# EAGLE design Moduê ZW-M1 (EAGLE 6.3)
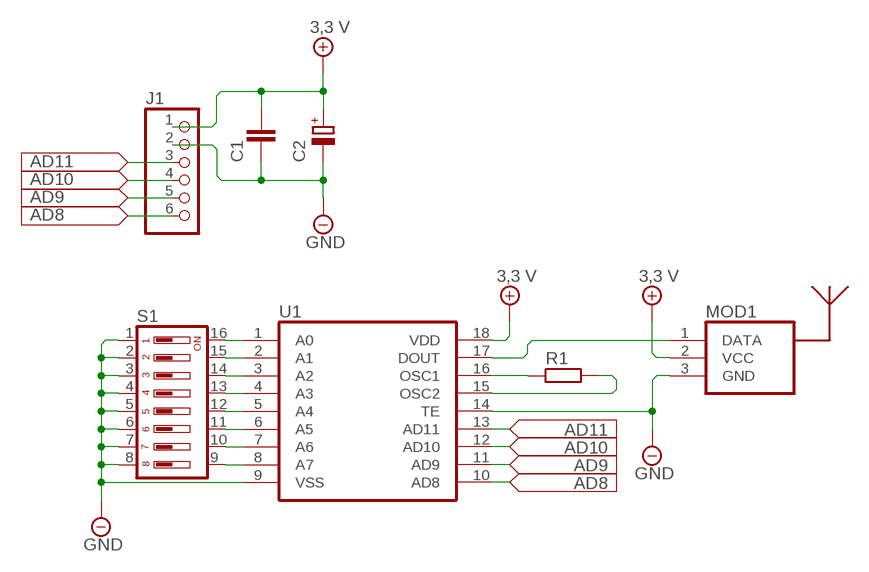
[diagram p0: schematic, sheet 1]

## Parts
C1  KONDENSATOR_CERAMICZNY  [KONDENSATOR_CERAMICZNY]
C2  KONDENSATOR_ELEKTROLITYCZNY_1  [KONDENSATOR_ELEKTROLITYCZNY_1]
J1  ZŁĄCZE_6_PIN  [ZŁĄCZE_6_PIN]
MOD1  NADAJNIK433MHZ  [NADAJNIK433MHZ]
R1  REZYSTOR  [REZYSTOR]
S1  DIP_SWITCH_8  [DIP_SWITCH_8]
U1  HT12F  [HT12F]

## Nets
5V: C1.1 C2.+ J1.1 MOD1.2(VCC) U1.18(VDD) ; supply symbol labelled 3,3 V
AD8: J1.6 U1.10(AD8)
AD9: J1.5 U1.11(AD9)
AD10: J1.4 U1.12(AD10)
AD11: J1.3 U1.13(AD11)
GND: C1.2 C2.- J1.2 MOD1.3(GND) S1.1 S1.2 S1.3 S1.4 S1.5 S1.6 S1.7 S1.8 U1.9(VSS) U1.14(TE)
N$18: S1.16 U1.1(A0)
N$22: S1.15 U1.2(A1)
N$23: S1.14 U1.3(A2)
N$24: S1.13 U1.4(A3)
N$25: S1.12 U1.5(A4)
N$26: S1.11 U1.6(A5)
N$27: S1.10 U1.7(A6)
N$28: S1.9 U1.8(A7)
N$29: R1.2 U1.15(OSC2)
N$30: R1.1 U1.16(OSC1)
N$35: MOD1.1(DATA) U1.17(DOUT)

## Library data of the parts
C1 = Własne:KONDENSATOR_CERAMICZNY
C2 = Własne:KONDENSATOR_ELEKTROLITYCZNY_1
J1 = Własne:ZŁĄCZE_6_PIN
MOD1 = Własne:NADAJNIK433MHZ
R1 = Własne:REZYSTOR
S1 = Własne:DIP_SWITCH_8
U1 = Własne:HT12F

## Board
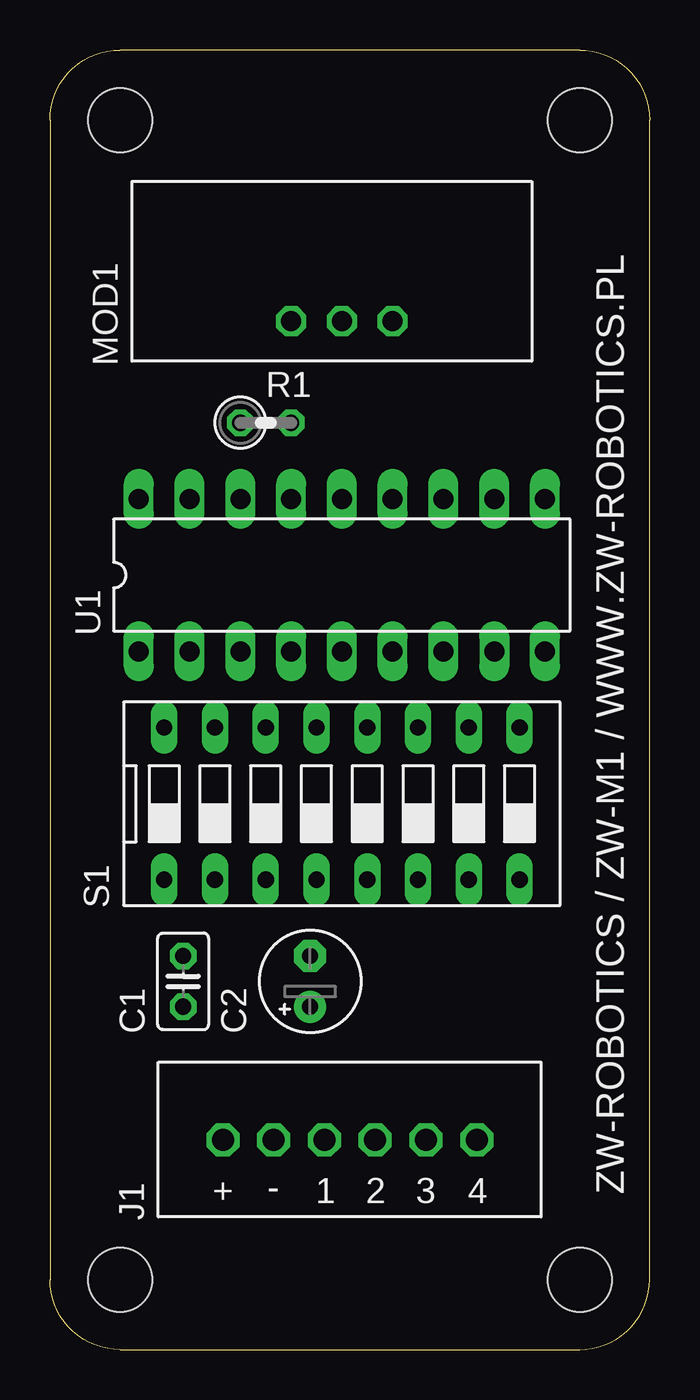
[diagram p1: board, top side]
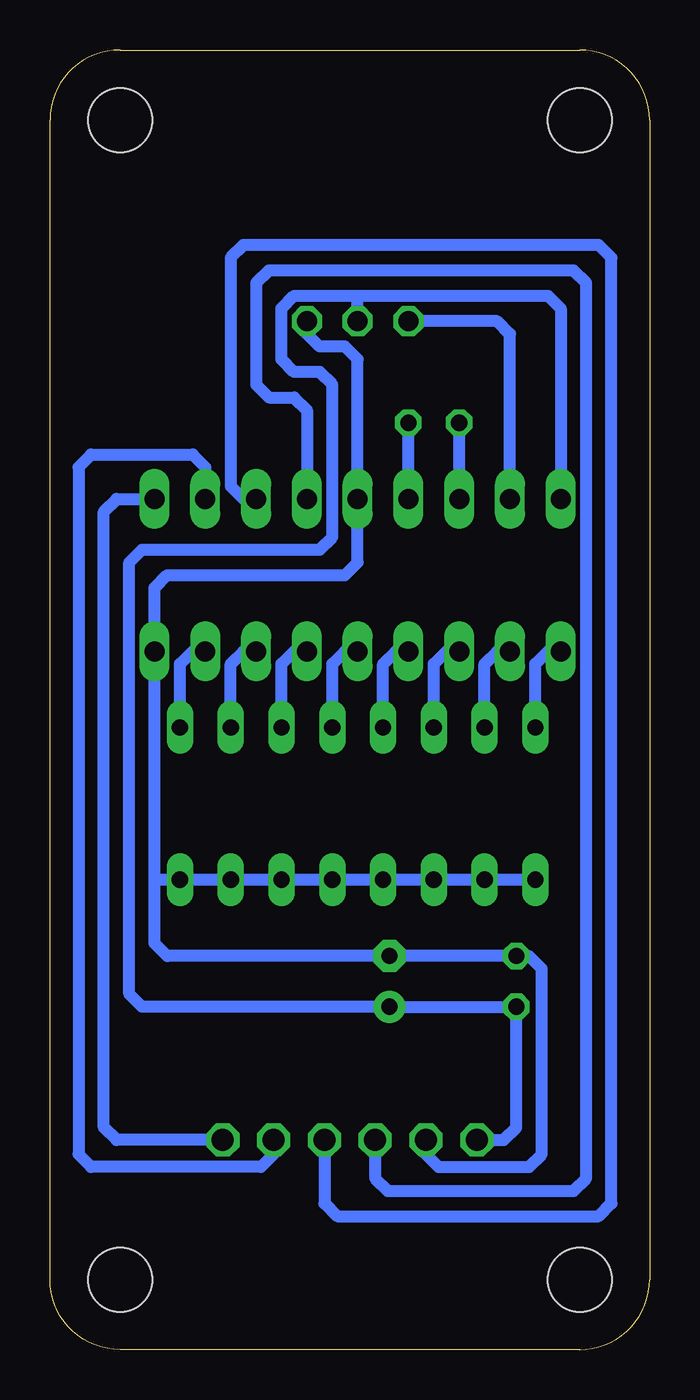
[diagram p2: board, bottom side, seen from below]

Size 30 x 65 mm. Coordinates in mm from the lower left corner, seen from the top.
Outline: 3.5,0 26.5,0 arc90 30,3.5 30,61.5 arc90 26.5,65 3.5,65 arc90 0,61.5 0,3.5 arc90 3.5,0
Copper layers (1*16): Top 0.035mm / dielectric 1.5mm / Bottom 0.035mm
Design rules "default": minimum track width 10mil, minimum drill 24mil, track to track 8mil, track to pad 8mil, pad to pad 8mil, via to via 8mil, smd to smd 8mil, copper to edge 40mil, drill to drill 8mil, minimum pad ring 10mil, minimum via ring 8mil, stop-mask expansion 4mil, vias tented up to drill 0mil, thermal gap 10mil
Holes 3.2 mm at 3.5,3.5 26.5,3.5 3.5,61.5 26.5,61.5

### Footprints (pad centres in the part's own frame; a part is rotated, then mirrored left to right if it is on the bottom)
KONDENSATOR_CERAMICZNY = drill 0.813 octagon: 1 -1.27,0; 2 1.27,0
KONDENSATOR_ELEKTROLITYCZNY_1 = drill 0.813 pad 1.6: + -1.27,0 | drill 0.813 pad 1.6 octagon: - 1.27,0
ZŁĄCZE_6_PIN = drill 1.1 octagon: 1 -6.35,0; 2 -3.81,0; 3 -1.27,0; 4 1.27,0; 5 3.81,0; 6 6.35,0
NADAJNIK433MHZ = drill 1 octagon: 1 -2.54,2.54; 2 -2.54,0; 3 -2.54,-2.54
REZYSTOR = drill 0.813 octagon: 1 -1.27,0; 2 1.27,0
DIP_SWITCH_8 = drill 0.813 long: 1 -8.89,-3.81; 2 -6.35,-3.81; 3 -3.81,-3.81; 4 -1.27,-3.81; 5 1.27,-3.81; 6 3.81,-3.81; 7 6.35,-3.81; 8 8.89,-3.81; 9 8.89,3.81; 10 6.35,3.81; 11 3.81,3.81; 12 1.27,3.81; 13 -1.27,3.81; 14 -3.81,3.81; 15 -6.35,3.81; 16 -8.89,3.81
HT12F = drill 1 long: 1 -10.16,-3.81; 2 -7.62,-3.81; 3 -5.08,-3.81; 4 -2.54,-3.81; 5 0,-3.81; 6 2.54,-3.81; 7 5.08,-3.81; 8 7.62,-3.81; 9 10.16,-3.81; 10 10.16,3.81; 11 7.62,3.81; 12 5.08,3.81; 13 2.54,3.81; 14 0,3.81; 15 -2.54,3.81; 16 -5.08,3.81; 17 -7.62,3.81; 18 -10.16,3.81

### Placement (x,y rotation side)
C1  6.67,18.41 90 top
C2  13.02,18.41 90 top
J1  15,10.48 0 top
MOD1  14.61,53.98 90 top
R1  10.79,46.35 0 top
S1  14.61,27.3 0 top
U1  14.61,38.73 0 top

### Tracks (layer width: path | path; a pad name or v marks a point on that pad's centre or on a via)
5V
  Bottom 0.61: J1.1 7.3,10.48 6.67,11.11 C1.1 C2.+ 25.4,17.14 26.04,17.78 26.04,39.37 25.4,40.01 16.51,40.01 15.88,40.64 15.88,48.26 16.51,48.9 17.78,48.9 18.41,49.53 18.41,52.07 17.78,52.7 14.61,52.7 | MOD1.2 14.61,52.7 | 14.61,52.7 5.08,52.7 4.45,52.07 U1.18
AD8
  Bottom 0.61: J1.6 26.67,10.48 27.3,11.11 27.3,41.91 26.67,42.55 U1.10
AD9
  Bottom 0.61: J1.5 18.81,9.77 19.45,9.13 27.94,9.13 28.57,9.77 28.57,44.13 27.94,44.77 22.86,44.77 22.23,44.13 U1.11
AD10
  Bottom 0.61: J1.4 16.27,7.3 15.63,6.67 2.54,6.67 1.91,7.3 1.91,54.61 2.54,55.24 20.32,55.24 20.95,54.61 20.95,43.18 20.32,42.55 U1.12
AD11
  Bottom 0.61: J1.3 13.73,8.57 13.1,7.94 3.81,7.94 3.17,8.57 3.17,53.34 3.81,53.98 19.05,53.98 19.68,53.34 19.68,48.26 19.05,47.62 17.78,47.62 17.14,46.99 U1.13
GND
  Bottom 0.61: J1.2 11.19,9.77 10.55,9.13 6.03,9.13 5.4,9.77 5.4,19.05 6.03,19.68 C1.2 C2.- 24.13,19.68 24.77,20.32 24.77,23.5 | 24.77,23.5 U1.9 24.77,38.1 24.13,38.73 15.24,38.73 14.61,39.37 U1.14 14.61,49.53 15.24,50.16 16.51,50.16 17.14,50.8 MOD1.3 | S1.1 S1.2 S1.3 S1.4 S1.5 S1.6 S1.7 S1.8 24.77,23.5
N$18
  Bottom 0.61: S1.16 5.71,34.29 5.08,34.92 U1.1
N$22
  Bottom 0.61: S1.15 8.26,34.29 7.62,34.92 U1.2
N$23
  Bottom 0.61: S1.14 10.79,34.29 10.16,34.92 U1.3
N$24
  Bottom 0.61: S1.13 13.34,34.29 12.7,34.92 U1.4
N$25
  Bottom 0.61: S1.12 15.88,34.29 15.24,34.92 U1.5
N$26
  Bottom 0.61: S1.11 18.41,34.29 17.78,34.92 U1.6
N$27
  Bottom 0.61: S1.10 20.95,34.29 20.32,34.92 U1.7
N$28
  Bottom 0.61: S1.9 23.5,34.29 22.86,34.92 U1.8
N$29
  Bottom 0.61: U1.15 R1.2
N$30
  Bottom 0.61: U1.16 R1.1
N$35
  Bottom 0.61: U1.17 6.99,50.8 7.62,51.44 MOD1.1

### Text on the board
tPlace: ZW-ROBOTICS / ZW-M1 / WWW.ZW-ROBOTICS.PL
